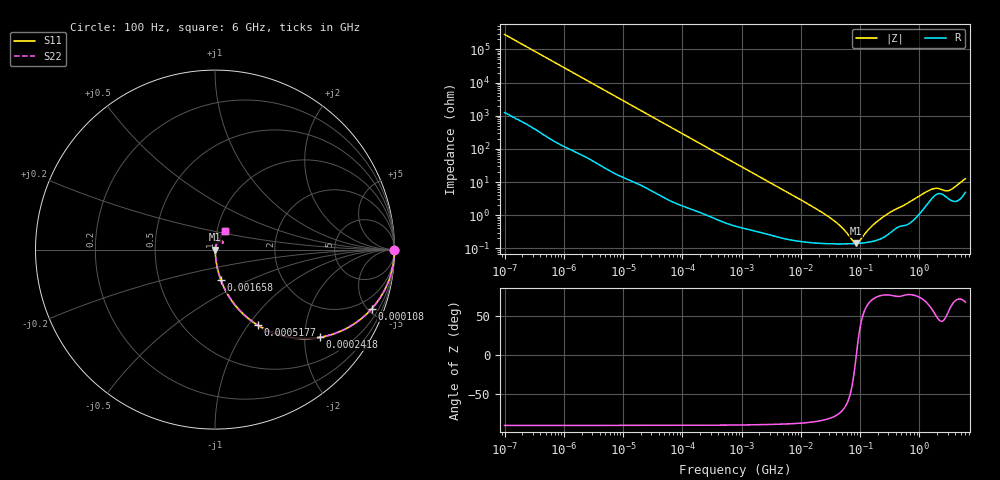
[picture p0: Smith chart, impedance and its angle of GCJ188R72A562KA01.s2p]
!Murata Part Number: GCJ188R72A562KA01
!These Parameters are Measured in Series Mode Connection
!Data Generated on Mar 13, 2026
!  o--ll--o
!Port1  Port2
!  o------o
!Operation Temp=25[degC], DC Bias Voltage=0[V]
!Freq. Start=100[Hz] Stop=6[GHz] 401[Steps]
# Hz S RI R 50
!Freq.(Hz) S11(Real) S11(Imag) S21(Real) S21(Imag) S12(Real) S12(Imag) S22(Real) S22(Imag)
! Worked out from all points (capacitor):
!   401 points, 100 Hz to 6 GHz, reference 50 ohm
!   read as one part in series: C = 5.67 nF near 109 Hz
!   lowest |Z| = 141 mohm at 85.28 MHz (marker M1)
!   series resonance near 86.5 MHz, so ESL is about 600 pH
!   S11 on the Smith chart (normalised r, x): 100 Hz: open; 108 kHz: 1.04, -5.30; 241.8 kHz: 1.02, -2.38; 517.7 kHz: 1.01, -1.11; 1.658 MHz: 1.01, -0.35; 6 GHz: 1.10, +0.23
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100  1 -0.000357  1.7e-06 0.000357  1.7e-06 0.000357  1 -0.000357
2008  0.9999 -0.0071  8.35e-05 0.0071  8.35e-05 0.0071  0.9999 -0.0071
12592  0.9978 -0.0442  0.00218 0.0442  0.00218 0.0442  0.9978 -0.0442
40335  0.9797 -0.1383  0.0203 0.1383  0.0203 0.1383  0.9797 -0.1383
108014  0.8737 -0.3288  0.1263 0.3288  0.1263 0.3288  0.8737 -0.3288
241822  0.5848 -0.4884  0.4152 0.4884  0.4152 0.4884  0.5848 -0.4884
517687  0.2393 -0.4213  0.7607 0.4213  0.7607 0.4213  0.2393 -0.4213
774597  0.1253 -0.3248  0.8747 0.3248  0.8747 0.3248  0.1253 -0.3248
1658239  0.0328 -0.1688  0.9672 0.1688  0.9672 0.1688  0.0328 -0.1688
4246196  0.00684 -0.0683  0.9932 0.0683  0.9932 0.0683  0.00684 -0.0683
1.555665e7  0.00182 -0.0184  0.9982 0.0184  0.9982 0.0184  0.00182 -0.0184
3.983537e7  0.0014 -0.00586  0.9986 0.00586  0.9986 0.00586  0.0014 -0.00586
5.449875e7  0.00138 -0.00328  0.9986 0.00328  0.9986 0.00328  0.00138 -0.00328
7.797396e7  0.00139 -0.000712  0.9986 0.000712  0.9986 0.000712  0.00139 -0.000712
8.527865e7  0.00141 -9.62e-05  0.9986 9.62e-05  0.9986 9.62e-05  0.00141 -9.62e-05
9.753859e7  0.00143 0.000829  0.9986 -0.000829  0.9986 -0.000829  0.00143 0.000829
1.669249e8  0.00167 0.00487  0.9983 -0.00487  0.9983 -0.00487  0.00167 0.00487
3.124326e8  0.00294 0.0115  0.9971 -0.0115  0.9971 -0.0115  0.00294 0.0115
1.497423e9  0.0284 0.048  0.9716 -0.048  0.9716 -0.048  0.0284 0.048
1.95892e9  0.0432 0.0447  0.9568 -0.0447  0.9568 -0.0447  0.0432 0.0447
3.065283e9  0.0327 0.0416  0.9673 -0.0416  0.9673 -0.0416  0.0327 0.0416
6e9  0.0583 0.1046  0.9417 -0.1046  0.9417 -0.1046  0.0583 0.1046
